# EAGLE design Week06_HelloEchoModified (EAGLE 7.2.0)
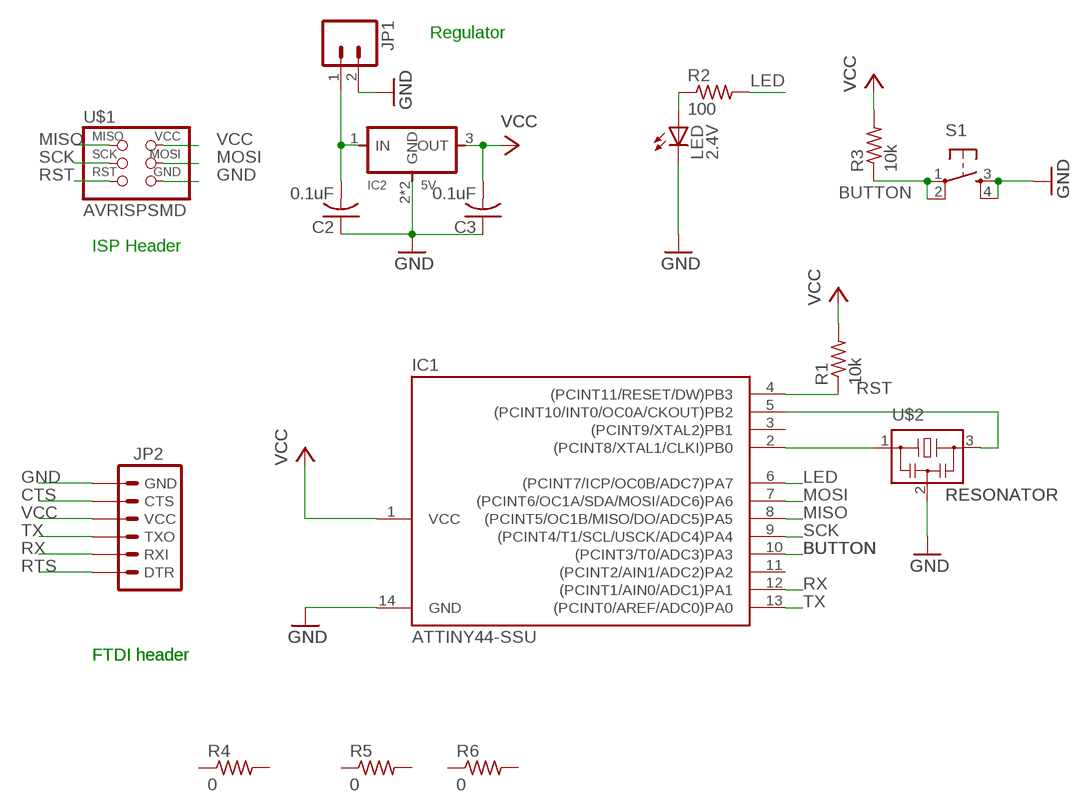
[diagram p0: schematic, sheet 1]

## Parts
C2  0.1uF  C-USC1206K  [C1206K]
C3  0.1uF  C-USC1206K  [C1206K]
IC1  ATTINY44-SSU  [SOIC14]
IC2  5V  REGULATORSOT223  [SOT223]
JP1  M02POLAR_LOCK  [MOLEX-1X2_LOCK]
JP2  ARDUINO_SERIAL_PROGRAMSMD  [1X06-SMD]
LED  2.4V  LED1206  [1206]
R1  10k  RESISTOR1206  [1206]
R2  100  R-US_R1206  [R1206]
R3  10k  R-US_R1206  [R1206]
R4  0  R-US_R1206  [R1206]
R5  0  R-US_M1206  [M1206]
R6  0  R-US_M1206  [M1206]
S1  6MM_SWITCH6MM_SWITCH  [6MM_SWITCH]
U$1  AVRISPSMD  [2X03SMD]
U$2  RESONATOR  [EFOBM]

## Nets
BUTTON: IC1.10((PCINT3/T0/ADC3)PA3) R3.1 S1.1(P) S1.2(P1)
CTS: JP2.5(CTS)
GND: C2.1 C3.1 IC1.14(GND) IC2.2(GND) IC2.4(GND) JP1.2 JP2.6(GND) LED.2(C) S1.3(S) S1.4(S1) U$1.6(GND) U$2.2
LED: IC1.6((PCINT7/ICP/OC0B/ADC7)PA7) R2.2
MISO: IC1.8((PCINT5/OC1B/MISO/DO/ADC5)PA5) U$1.1(MISO)
MOSI: IC1.7((PCINT6/OC1A/SDA/MOSI/ADC6)PA6) U$1.4(MOSI)
N$1: LED.1(A) R2.1
N$2: C2.2 IC2.1(IN) JP1.1
N$6: IC1.5((PCINT10/INT0/OC0A/CKOUT)PB2) U$2.3
RESONATOR: IC1.2((PCINT8/XTAL1/CLKI)PB0) U$2.1
RST: IC1.4((PCINT11/RESET/DW)PB3) R1.1 U$1.5(RST)
RTS: JP2.1(DTR)
RX: IC1.12((PCINT1/AIN0/ADC1)PA1) JP2.2(RXI)
SCK: IC1.9((PCINT4/T1/SCL/USCK/ADC4)PA4) U$1.3(SCK)
TX: IC1.13((PCINT0/AREF/ADC0)PA0) JP2.3(TXO)
VCC: C3.2 IC1.1(VCC) IC2.3(OUT) JP2.4(VCC) R1.2 R3.2 U$1.2(VCC)
Unconnected: IC1.3((PCINT9/XTAL2)PB1) IC1.11((PCINT2/AIN1/ADC2)PA2) R4.1 R4.2 R5.1 R5.2 R6.1 R6.2

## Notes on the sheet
- Regulator
- ISP Header
- FTDI header | FTDI header

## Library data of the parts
C2 C3 = 01_adafruit:C-US: CAPACITOR, American symbol
IC1 = 01_FAB_Hello:ATTINY44
IC2 = 01_fab:REGULATOR
JP1 = 01_SparkFun:M02: Header 2
JP2 = SparkFun-Connectors:ARDUINO_SERIAL_PROGRAM: FTDI connector footprints; PROD_ID: CONN-08971
LED = 01_FAB_Hello:LED
R1 = 01_FAB_Hello:RESISTOR
R2-R6 = 01_adafruit:R-US_: RESISTOR, American symbol
S1 = 01_FAB_Hello:6MM_SWITCH: OMRON SWITCH
U$1 = fab:AVRISP
U$2 = fab:RESONATOR

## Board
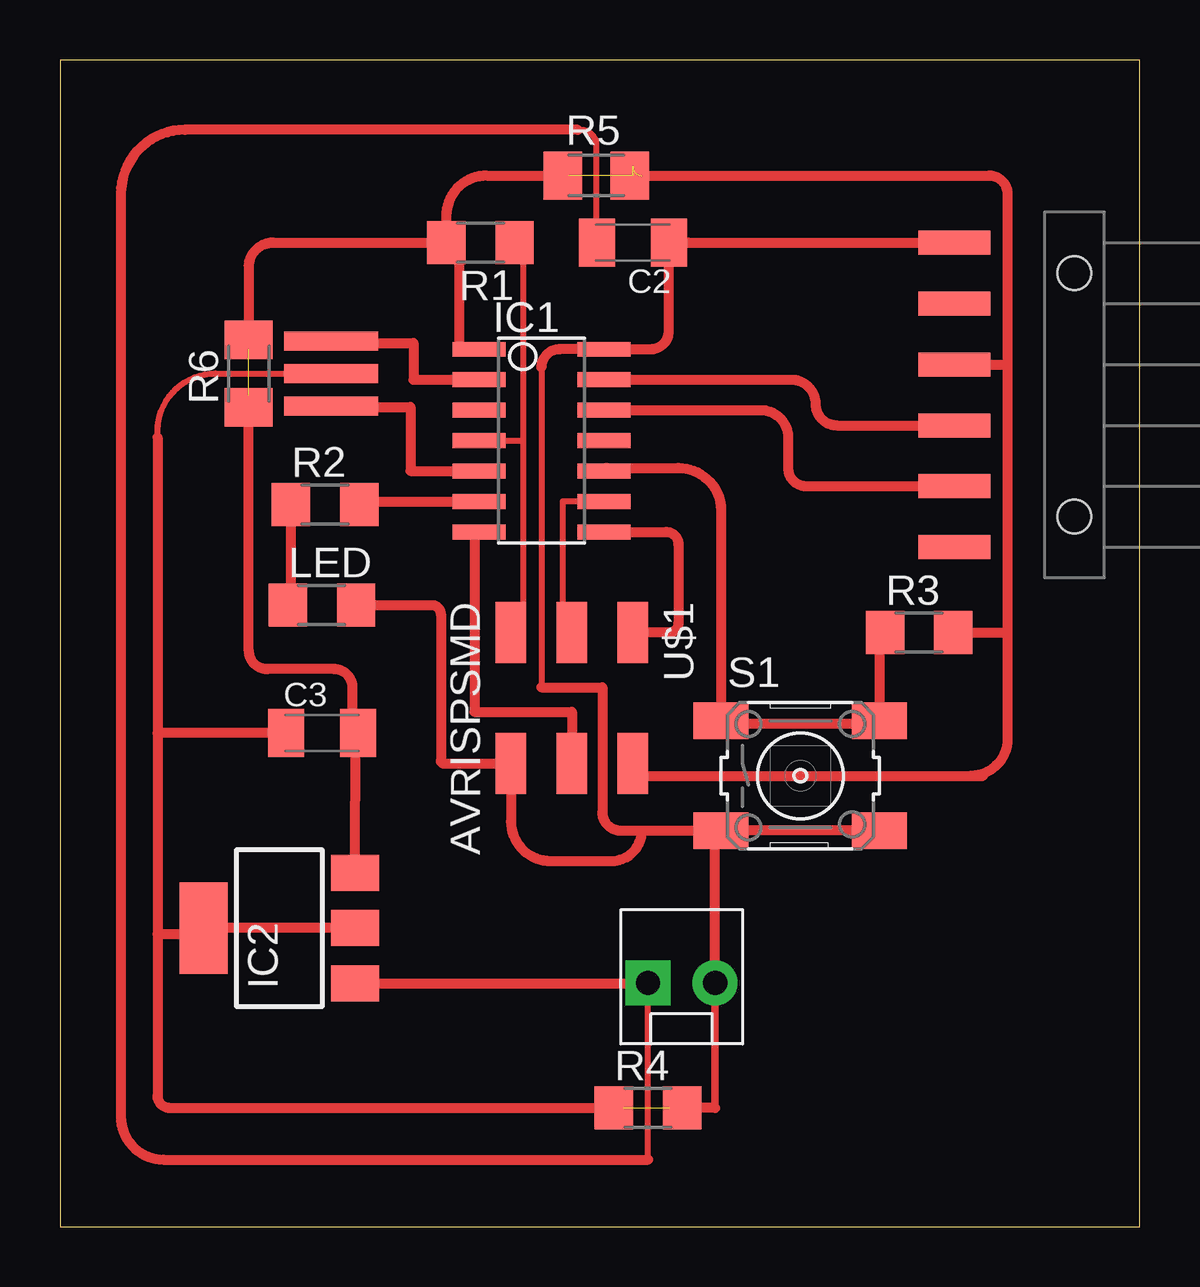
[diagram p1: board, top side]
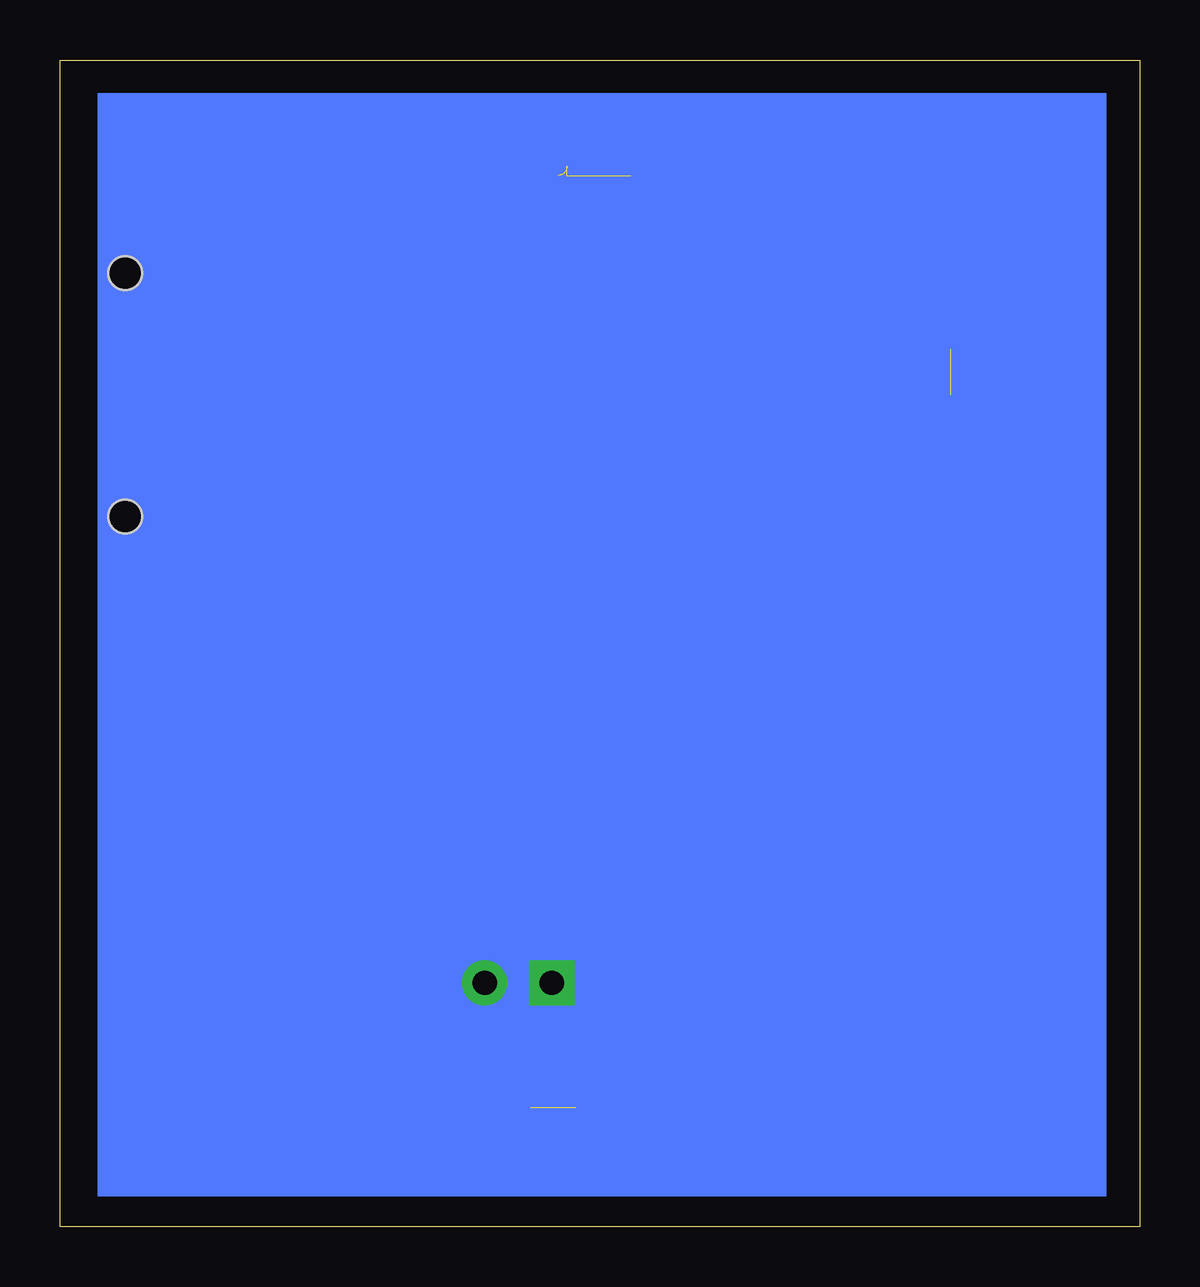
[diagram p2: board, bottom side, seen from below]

Size 45.01 x 48.63 mm. Coordinates in mm from the lower left corner, seen from the top.
Outline: 0,0 45.01,0 45.01,48.63 0,48.63 0,0
Copper layers (1*16): Top 0.035mm / dielectric 1.5mm / Bottom 0.035mm
Design rules "fabmodule": minimum track width 10mil, minimum drill 0.4mm, track to track 0.42mm, track to pad 0.42mm, pad to pad 0.42mm, via to via 0.42mm, smd to smd 0.42mm, copper to edge 40mil, drill to drill 0.8mm, minimum pad ring 10mil, minimum via ring 8mil, stop-mask expansion 4mil, vias tented up to drill 0mil, thermal gap 10mil

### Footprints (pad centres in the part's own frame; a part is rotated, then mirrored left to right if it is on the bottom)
C1206K = smd 1.5 x 2: 1 -1.5,0; 2 1.5,0
SOIC14 = smd 0.61 x 2.21: 1 -3.81,-2.603; 2 -2.54,-2.603; 3 -1.27,-2.603; 4 0,-2.603; 5 1.27,-2.603; 6 2.54,-2.603; 7 3.81,-2.603; 8 3.81,2.603; 9 2.54,2.603; 10 1.27,2.603; 11 0,2.603; 12 -1.27,2.603; 13 -2.54,2.603; 14 -3.81,2.603
SOT223 = smd 1.5 x 2: 1 -2.3,-3.15; 2 0,-3.15; 3 2.3,-3.15 | smd 3.8 x 2: 4 0,3.15
MOLEX-1X2_LOCK = drill 1.016 pad 1.88 square: 1 -0.127,0 | drill 1.016 pad 1.88: 2 2.667,0
1X06-SMD = smd 1 x 3: 1 -6.35,5; 2 -3.81,5; 3 -1.27,5; 4 1.27,5; 5 3.81,5; 6 6.35,5 | hole 1.4: -5.08,0; 5.08,0
1206 = smd 1.6 x 1.803: 1 -1.422,0; 2 1.422,0
R1206 = smd 1.6 x 1.803: 1 -1.422,0; 2 1.422,0
M1206 = smd 1.6 x 2: 1 -1.4,0; 2 1.4,0
6MM_SWITCH = smd 2.286 x 1.524: 1 -3.302,2.286; 2 3.302,2.286; 3 -3.302,-2.286; 4 3.302,-2.286
2X03SMD = smd 2.54 x 1.27: 1 -2.54,2.54; 2 2.92,2.54; 3 -2.54,0; 4 2.92,0; 5 -2.54,-2.54; 6 2.92,-2.54
EFOBM = smd 0.8 x 3.9: 1 -1.35,0; 2 0,0; 3 1.35,0

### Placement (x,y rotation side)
C2  23.88,41.02 180 top
C3  10.92,20.57 0 top
IC1  20.07,32.77 270 top
IC2  9.14,12.45 90 top
JP1  24.64,10.16 0 top
JP2  42.29,34.67 90 top
LED  10.92,25.91 0 top
R1  17.53,41.02 180 top
R2  11.05,30.1 0 top
R3  35.81,24.77 0 top
R4  24.51,4.95 0 top
R5  22.35,43.81 0 top
R6  7.87,35.56 90 top
S1  30.86,18.8 0 top
U$1  21.34,22.23 270 top
U$2  11.3,35.56 270 top

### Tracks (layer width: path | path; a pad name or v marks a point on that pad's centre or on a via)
BUTTON
  Top 0.406: R3.1 arc90 34.16,24.54 S1.2 arc-90 34.04,20.95 27.69,20.95 arc-90 S1.1 27.56,29.84 arc90 25.78,31.62 22.8,31.62 arc90 IC1.10
GND  (1 unrouted)
  Top 0.254: 4.06,32.89 4.06,33.15 arc-90 6.48,35.56 U$2.2 | 20.07,35.81 20.07,22.48
  Top 0.305: C2.1 arc-90 25.78,40.62 | 27.3,4.95 27.3,9.52
  Top 0.406: 20.07,35.81 arc-90 20.83,36.58 IC1.14 24.64,36.58 arc90 25.38,37.31 C2.1 | 24.26,16.51 23.37,16.51 arc-90 22.61,17.27 22.61,22.48 20.07,22.48 | 24.26,16.51 S1.3 | 25.78,40.62 arc-90 26.19,41.02 JP2.6 | S1.4 S1.3 | IC2.2 IC2.4 arc-90 5.74,12.19 4.06,12.19 | 4.06,32.89 4.06,20.57 | 4.06,20.57 4.06,12.19 | 27.3,9.52 JP1.2 27.3,16.38 | 27.3,16.38 27.3,17.02 | LED.2 15.49,25.91 arc-90 15.88,25.53 15.88,19.43 arc90 16,19.3 U$1.6 18.8,16.89 arc90 20.45,15.24 22.99,15.24 arc90 24.26,16.51 | C3.1 4.06,20.57 | 4.06,12.19 4.06,5.46 arc90 4.57,4.95 23.5,4.95 | S1.3 arc-90 27.43,16.38 27.3,16.38 | 27.3,4.95 25.4,4.95
LED
  Top 0.406: R2.2 arc-90 12.6,30.23 IC1.6
MISO
  Top 0.406: IC1.8 25.27,28.96 arc-90 25.78,28.45 25.78,25.15 arc-90 25.4,24.77 U$1.1
MOSI
  Top 0.406: IC1.7 arc90 17.27,28.77 17.27,21.46 21.34,21.46 U$1.4
N$1
  Top 0.406: LED.1 arc90 9.63,26.03 R2.1
N$2
  Top 0.254: 21.59,45.72 21.72,45.72 arc-90 22.35,45.08 22.35,41.05 arc90 C2.2 | 24.51,2.79 JP1.1
  Top 0.406: 21.59,45.72 5.21,45.72 arc90 2.54,43.05 2.54,4.57 arc90 4.32,2.79 24.51,2.79 | IC2.1 24.5,10.15 arc90 JP1.1 | C2.2 arc-90 22.35,41.05 arc90 C2.2
N$6
  Top 0.406: U$2.3 arc90 11.35,34.16 14.61,34.16 14.61,31.5 IC1.5
RESONATOR
  Top 0.406: U$2.1 arc90 11.38,36.83 14.73,36.83 14.73,35.31 IC1.2
RST
  Top 0.254: 19.3,40.54 19.3,32.77 | 19.3,32.77 19.3,25.27 arc90 18.8,25.27 U$1.5 | IC1.4 19.3,32.77
  Top 0.305: R1.1 arc-90 19.24,40.54
  Top 0.406: 19.24,40.54 19.3,40.54
RX
  Top 0.406: IC1.12 29.21,34.04 arc-90 30.35,32.89 30.35,31.62 arc90 31.11,30.86 JP2.2
SCK
  Top 0.254: IC1.9 20.96,30.23 20.96,25.78 arc-90 21.34,25.53 U$1.3
TX
  Top 0.406: IC1.13 30.48,35.31 arc-90 31.5,34.29 arc90 32.38,33.4 JP2.3
VCC  (5 unrouted)
  Top 0.254: 12.32,20.71 12.32,20.68 arc90 C3.2
  Top 0.406: R1.2 16.64,41.02 16.64,36.58 IC1.1 | U$1.2 arc90 24.39,18.8 37.97,18.8 | 37.97,18.8 38.48,18.8 | R1.2 16.1,42.14 arc-90 17.78,43.81 21.21,43.81 | IC2.3 12.32,20.71 arc90 12.45,20.84 12.45,21.34 | 12.83,20.57 C3.2 arc-90 12.19,20.8 12.19,22.48 arc90 11.43,23.24 8.64,23.24 arc-90 7.87,24 7.87,34.67 | R1.2 8.89,41.02 arc90 7.87,40 7.87,36.58 | 23.5,43.81 38.73,43.81 arc-90 39.5,43.05 39.5,35.81 | 39.5,35.81 39.5,24.77 | 39.5,24.77 39.5,20.32 arc-90 37.97,18.8 | JP2.4 39.37,35.94 arc-90 39.5,35.81 | R3.2 39.5,24.77
(copper drawn outside any net)
  shapes: Bottom area x1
